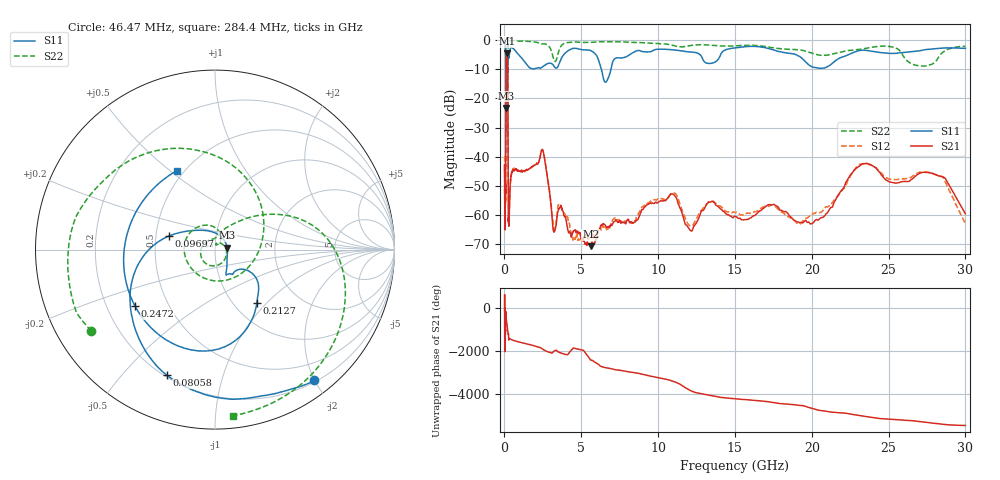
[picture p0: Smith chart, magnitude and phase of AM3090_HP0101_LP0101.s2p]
! Date/Time: Thu, Feb 28, 2019 1:58 PM
! Network Analyzer: Agilent Technologies E8364B Rev: A.07.50.67
! Sweep from 0.010 to 30.000 GHz, 1601 Points, Sweep Type: LOG
! Power Supply: 5.023 V, 0.002 A
# Hz S DB R 50
!freq MagS11 AngS11 MagS21 AngS21 MagS12 AngS12 MagS22 AngS22
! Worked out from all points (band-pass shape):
!   1601 points, 10 MHz to 30 GHz, reference 50 ohm
!   highest |S21| = -4.54 dB at 148.4 MHz (marker M1); lowest = -70.7 dB at 5.612 GHz (marker M2)
!   |S21| within 3 dB of the highest: 107.1 MHz to 202.1 MHz (94.99 MHz wide, 61.4 % of centre)
!   lowest |S11| = -23.3 dB at 105.1 MHz (marker M3), VSWR 1.15, Z = 57.3 + j1.24 ohm
!   |S11| at or under -10 dB: 96.09 MHz to 203.3 MHz (107.2 MHz wide, 71.6 % of centre); 6.308 GHz to 6.932 GHz (624 MHz wide, 9.43 % of centre)
!   |S22| runs from -31.6 to -0.1 dB; largest |S21 - S12| = 0.015
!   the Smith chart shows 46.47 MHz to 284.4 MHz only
!   S11 on the Smith chart (normalised r, x): 46.47 MHz: 0.22, -1.99; 80.58 MHz: 0.21, -0.67; 96.97 MHz: 0.58, +0.09; 212.7 MHz: 1.26, -0.88; 247.2 MHz: 0.32, -0.29; 284.4 MHz: 0.46, +0.53
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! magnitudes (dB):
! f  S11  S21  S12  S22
! 10 MHz  -0.3  -45.3  -39.8  -0.5
! 38.04 MHz  -0.5  -61.8  -59.9  -1.4
! 46.47 MHz  -0.8  -51.0  -48.5  -1.7
! 80.58 MHz  -2.5  -48.9  -49.9  -5.0
! 96.97 MHz  -11.4  -15.9  -15.9  -15.3
! 105.1 MHz  -23.3  -8.3  -8.3  -15.5
! 130.3 MHz  -16.2  -4.8  -4.8  -31.6
! 144.7 MHz  -16.2  -4.6  -4.5  -25.2
! 148.4 MHz  -16.0  -4.5  -4.5  -23.9
! 212.7 MHz  -8.4  -11.4  -11.3  -12.6
! 247.2 MHz  -5.3  -56.4  -55.8  -1.5
! 284.4 MHz  -6.2  -63.7  -61.4  -0.6
! 550.5 MHz  -2.9  -44.4  -44.3  -0.2
! 2.084 GHz  -9.7  -42.5  -42.3  -0.8
! 2.545 GHz  -8.9  -38.8  -38.7  -1.3
! 3.236 GHz  -9.1  -65.8  -65.0  -7.1
! 5.612 GHz  -3.6  -70.7  -67.4  -0.8
! 6.619 GHz  -14.4  -63.9  -64.5  -0.6
! 7.926 GHz  -5.7  -62.2  -62.5  -0.7
! 19.9 GHz  -8.9  -63.0  -60.0  -4.3
! 23.59 GHz  -3.6  -42.2  -42.5  -2.8
! 30 GHz  -2.9  -59.5  -62.9  -2.2
